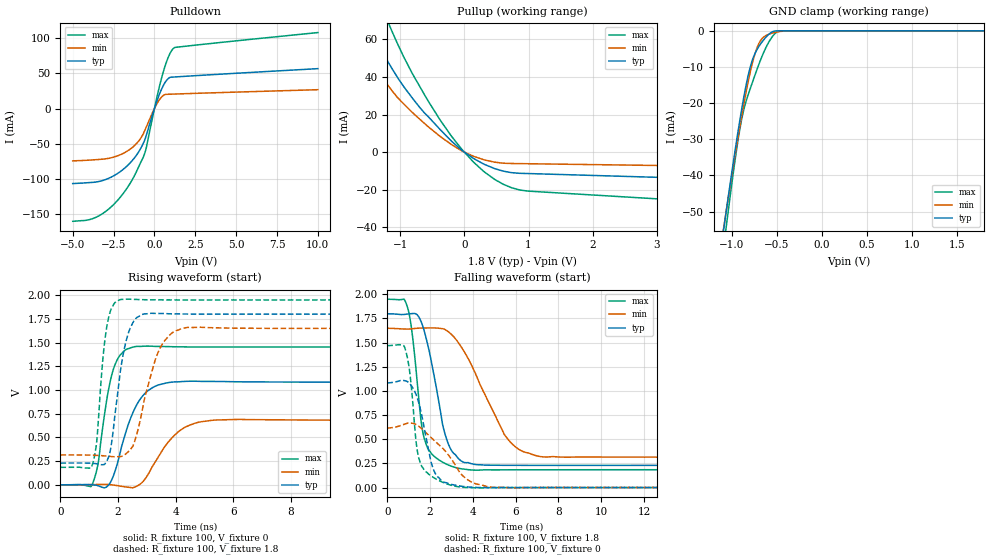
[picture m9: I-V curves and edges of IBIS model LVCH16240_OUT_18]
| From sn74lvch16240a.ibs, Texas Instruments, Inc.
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[Model]   LVCH16240_OUT_18
Model_type  3-state
Enable   Active-Low
Vref =   0
Rref =   500
Cref =   30p
Vmeas =   0.9
| variable   typ   min   max
C_comp   5.02pF   4.61pF   6.05pF
| C_pullup   8.43pF   3.38pF   19.51pF
| C_pulldown   8.31pF   5.63pF   10.77pF
| C_tri-state   5.02pF   4.61pF   6.05pF
[Temperature Range]   40   100   -40
| Ambient temperature   25   85   -40
[Voltage range]   1.8   1.65   1.95
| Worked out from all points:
|   slope of the pulldown table from 0 to 0.27 V, typ, clamps not added: 14.8 ohm
|   slope of the pullup table from 0 to 0.27 V, typ, clamps not added: 46.7 ohm
|   GND clamp passes 1 mA (typ) near -0.59 V on its own axis
|   rising waveform, R_fixture 100, V_fixture 0: 20-80 % time 724ps typ, 945ps min, 446ps max; typ from 0 V to 1.09 V
|   falling waveform, R_fixture 100, V_fixture 1.8: 20-80 % time 829ps typ, 1.74ns min, 533ps max; typ from 1.8 V to 0.23 V
|   rising waveform, R_fixture 100, V_fixture 1.8: 20-80 % time 434ps typ, 678ps min, 291ps max; typ from 0.23 V to 1.8 V
|   falling waveform, R_fixture 100, V_fixture 0: 20-80 % time 628ps typ, 1.35ns min, 428ps max; typ from 1.08 V to 0 V
[GND Clamp]
| LVCH16240_OUT_18
|   Voltage   I(typ)   I(min)   I(max)
-5V       -855.7mA   -797.6mA   -953.2mA
-1.085V   -53.47mA   -53.15mA   -58.22mA
-1.06V    -49.06mA   -49.09mA   -53.29mA
-975mV    -34.56mA   -35.69mA   -37.29mA
-910mV    -24.24mA   -26.03mA   -26.76mA
-865mV    -17.79mA   -19.78mA   -21.4mA
-800mV    -10.27mA   -11.72mA   -16.17mA
-740mV    -6.037mA   -5.97mA    -11.9mA
-685mV    -3.711mA   -2.772mA   -8.196mA
-590mV    -945.4uA   -940.9uA   -3.072mA
-510mV    -31.84uA   -379.7uA   -498.3uA
1.8V      7.564pA    17.59nA    -112.7pA
[Pulldown]
| LVCH16240_OUT_18
|   Voltage   I(typ)   I(min)   I(max)
-5V       -106.8mA   -74.48mA   -160.5mA
-3.945V   -105.3mA   -73.35mA   -157.9mA
-3.11V    -102mA     -71.9mA    -148.6mA
-2.21V    -91.71mA   -66.9mA    -129.5mA
-1.4V     -75.15mA   -56.3mA    -103.1mA
-920mV    -59.95mA   -44.93mA   -80.72mA
-585mV    -44.32mA   -30.88mA   -63.04mA
60mV      4.341mA    2.845mA    6.529mA
455mV     28.54mA    16.86mA    44.89mA
845mV     42.74mA    20.36mA    72.96mA
1.185V    44.91mA    20.64mA    86.07mA
10V       56.83mA    26.86mA    108.2mA
[Pullup]
| LVCH16240_OUT_18
|   Voltage   I(typ)   I(min)   I(max)
-5V       29.31mA    10.34mA    78.9mA
-3.56V    38.96mA    11.4mA     214.8mA
-3.24V    48.87mA    12.22mA    244.5mA
-3.11V    69.83mA    12.77mA    236.3mA
-2.795V   142.2mA    15.56mA    212.5mA
-2.62V    134.9mA    22.74mA    198mA
-2.515V   129.6mA    70.32mA    189mA
-1.885V   92.49mA    69.08mA    132.8mA
-1.13V    44.7mA     32.87mA    64.59mA
-35mV     915.1uA    617uA      1.397mA
860mV     -11.22mA   -6.065mA   -20.08mA
10V       -20.36mA   -10.29mA   -39.14mA
[Ramp]
| LVCH16240_OUT_18
| variable   typ   min   max
dV/dt_r   0.67/7.72E-10   0.43/1.02E-09   0.89/4.60E-10
dV/dt_f   0.94/9.22E-10   0.80/1.79E-09   1.06/5.80E-10
R_load = 100
[Rising Waveform]
| LVCH16240_OUT_18
R_fixture =   100
C_fixture =   0
L_fixture =   0
V_fixture =   0
V_fixture_min = 0
V_fixture_max = 0
|   Time   V(typ)   V(min)   V(max)
0s        -7.073uV   -11.38uV   46.27uV
1.085ns   710.2uV    1.965mV    -6.325mV
1.305ns   -10.42mV   3.205mV    220.4mV
1.62ns    -17.83mV   3.17mV     921.3mV
1.84ns    96.39mV    -3.006mV   1.221V
2.635ns   837.2mV    -17.1mV    1.459V
3.22ns    1.029V     207mV      1.461V
4.08ns    1.086V     556mV      1.455V
5.435ns   1.09V      684.2mV    1.453V
49.99ns   1.085V     680.4mV    1.454V
[Falling Waveform]
| LVCH16240_OUT_18
R_fixture =   100
C_fixture =   0
L_fixture =   0
V_fixture =   1.8
V_fixture_min = 1.65
V_fixture_max = 1.95
|   Time   V(typ)   V(min)   V(max)
0s        1.799V     1.649V     1.949V
950ps     1.796V     1.64V      1.862V
1.185ns   1.801V     1.644V     1.557V
1.52ns    1.747V     1.65V      813.4mV
1.89ns    1.48V      1.652V     406.5mV
2.705ns   549.5mV    1.634V     248.5mV
3.445ns   276.7mV    1.459V     194.8mV
5.515ns   230mV      534.8mV    183.2mV
7.235ns   229.3mV    318.1mV    184mV
49.99ns   229.5mV    315.1mV    184mV
[Rising Waveform]
| LVCH16240_OUT_18
R_fixture =   100
C_fixture =   0
L_fixture =   0
V_fixture =   1.8
V_fixture_min = 1.65
V_fixture_max = 1.95
|   Time   V(typ)   V(min)   V(max)
0s        229.5mV    314.9mV    184mV
1.095ns   226.8mV    312.2mV    202.8mV
1.25ns    222.4mV    310.4mV    428.7mV
1.465ns   211.9mV    306.5mV    1.303V
1.615ns   254mV      303mV      1.679V
2.115ns   1.268V     299.1mV    1.956V
2.65ns    1.764V     533.5mV    1.955V
3.435ns   1.807V     1.427V     1.95V
4.41ns    1.801V     1.66V      1.95V
49.99ns   1.799V     1.649V     1.949V
[Falling Waveform]
| LVCH16240_OUT_18
R_fixture =   100
C_fixture =   0
L_fixture =   0
V_fixture =   0
V_fixture_min = 0
V_fixture_max = 0
|   Time   V(typ)   V(min)   V(max)
0s        1.083V     615.5mV    1.469V
860ps     1.103V     659.5mV    1.417V
1.07ns    1.07V      667.7mV    1.157V
1.37ns    948mV      649mV      433.8mV
1.595ns   763.8mV    611.3mV    226.9mV
2.24ns    146.5mV    477.5mV    93.31mV
3.38ns    16.43mV    158.4mV    6.021mV
4.145ns   1.23mV     38.16mV    -2.714mV
5.85ns    227.6uV    -2.339mV   -17.67uV
49.99ns   20.92uV    50.24uV    55.17uV
